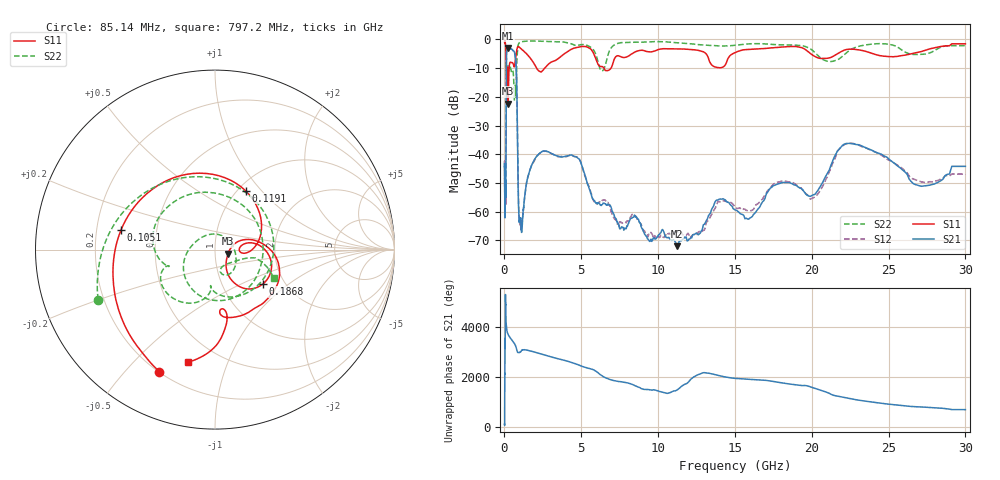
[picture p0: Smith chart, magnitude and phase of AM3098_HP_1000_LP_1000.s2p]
! Date/Time: Thu, Feb 28, 2019 8:40 AM
! Network Analyzer: Agilent Technologies E8364B Rev: A.07.50.67
! Sweep from 0.010 to 30.000 GHz, 1601 Points, Sweep Type: LOG
! Power Supply: 5.023 V, 0.002 A
# Hz S DB R 50
!freq MagS11 AngS11 MagS21 AngS21 MagS12 AngS12 MagS22 AngS22
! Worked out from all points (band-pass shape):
!   1601 points, 10 MHz to 30 GHz, reference 50 ohm
!   highest |S21| = -2.98 dB at 242.3 MHz (marker M1); lowest = -72.0 dB at 11.25 GHz (marker M2)
!   |S21| within 3 dB of the highest: 128 MHz to 706.1 MHz (578.1 MHz wide, 139 % of centre)
!   lowest |S11| = -22.3 dB at 239.9 MHz (marker M3), VSWR 1.17, Z = 57.9 - j2.54 ohm
!   |S11| at or under -10 dB: 191.2 MHz to 303.6 MHz (112.4 MHz wide, 45.4 % of centre); 2.093 GHz to 2.622 GHz (528.9 MHz wide, 22.4 % of centre); 6.482 GHz to 6.934 GHz (452.1 MHz wide, 6.74 % of centre)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
!   |S22| runs from -21.3 to -0.5 dB; largest |S21 - S12| = 0.014
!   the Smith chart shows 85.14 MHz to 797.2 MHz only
!   S11 on the Smith chart (normalised r, x): 85.14 MHz: 0.20, -0.62; 105.1 MHz: 0.31, +0.09; 119.1 MHz: 1.08, +0.82; 186.8 MHz: 1.55, -0.67; 797.2 MHz: 0.34, -0.73
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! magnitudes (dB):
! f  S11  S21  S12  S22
! 10 MHz  -0.4  -44.5  -42.8  -0.6
! 38.04 MHz  -0.5  -59.2  -57.9  -0.9
! 85.14 MHz  -2.5  -55.0  -54.4  -3.0
! 105.1 MHz  -5.4  -27.2  -27.0  -7.0
! 119.1 MHz  -8.6  -10.2  -10.2  -9.9
! 144.7 MHz  -16.7  -4.2  -4.1  -12.9
! 186.8 MHz  -9.7  -3.5  -3.5  -8.9
! 239.9 MHz  -22.3  -3.0  -2.9  -11.3
! 242.3 MHz  -22.1  -3.0  -2.9  -11.2
! 550.5 MHz  -8.3  -3.9  -3.8  -11.0
! 655.8 MHz  -9.3  -4.5  -4.5  -21.3
! 797.2 MHz  -3.8  -15.6  -15.6  -8.8
! 921.7 MHz  -2.5  -58.9  -57.6  -1.5
! 1.044 GHz  -3.1  -62.6  -64.9  -0.9
! 2.084 GHz  -9.9  -40.8  -40.8  -0.6
! 4.734 GHz  -2.8  -41.1  -41.0  -2.1
! 6.36 GHz  -9.4  -57.5  -56.1  -11.0
! 7.926 GHz  -6.2  -65.9  -63.9  -1.0
! 11.25 GHz  -3.3  -72.0  -67.2  -1.2
! 20.1 GHz  -5.6  -54.1  -55.2  -4.1
! 22.56 GHz  -3.4  -36.3  -36.2  -3.5
! 30 GHz  -1.5  -44.2  -46.9  -2.2
